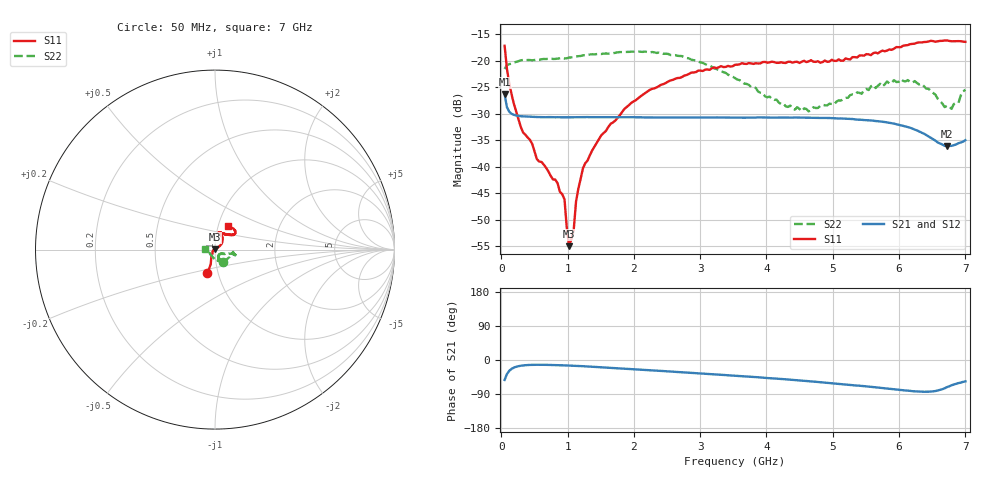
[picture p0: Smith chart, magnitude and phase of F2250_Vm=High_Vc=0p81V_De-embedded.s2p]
! Integrated Device Technology
! Corporate Headquarters
! 6024 Silver Creek Valley Road
! San Jose, CA 95138  USA
! Phone:  1-408-284-8200
! Toll Free:  1-800-223-1366
! Webpage:  http://www.idt.com/
! Timing and RF Division
! 515 Groton Road, Suite 102
! Westford, MA 01886-6024
! Device:  F2250
! Description: Voltage Variable RF Attenuator
! Frequency:  50.0 -  6000.00 MHz
! Package:  3x3 mm Thin QFN Plastic Package: 16 pin
! Ports:  2 RF, 3 DC
!  Pin  1  = GND
!  Pin  2  = NC
!  Pin  3  = RF1  = Port 1
!  Pin  4  = NC
!  Pin  5  = GND
!  Pin  6  = GND
!  Pin  7  = GND
!  Pin  8  = GND
!  Pin  9  = NC
!  Pin 10  = RF2  = Port 2
!  Pin 11  = NC
!  Pin 12  = GND
!  Pin 13  = GND
!  Pin 14  = VCNTRL
!  Pin 15  = VDD
!  Pin 16  = VMODE
! Vcntrl:  0.810 Volts
! Vmode:  +3.300 Volts
! Vdd:  +3.30  Volts
! Current:  1.304 mA
! Data:  The device was measured on a the F2250 evaluation board which has
!  individual transmission lines to the RF pins.  Data was collected
!  using a calibrated network analyzer.  The evaluation board was
!  de-embedded using a TRL calibration technique.
!  The reference plane is the edge of the package pin.
! Misc:  SN 10
!  Action Tracker AT0258
! Date Measured:  2014-11-26
! Date:  2015-10-15  MJV
! Note:
!  Integrated Device Technology supplies this data as a sample of measured
!  data at the package pin for this product.  Your particular data for this
!  product may vary.
!  Data was taken at 25 degrees C.
!  Integrated Device Technology reserves the right to change this data at anytime.
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# GHz S dB R 50
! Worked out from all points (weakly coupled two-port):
!   201 points, 50 MHz to 7 GHz, reference 50 ohm
!   highest |S21| = -26.31 dB at 50 MHz (marker M1); lowest = -36.1 dB at 6.722 GHz (marker M2)
!   lowest |S11| = -55.0 dB at 1.023 GHz (marker M3), VSWR 1.00, Z = 49.9 + j0.141 ohm
!   |S11| at or under -10 dB: start of sweep to end of sweep
!   |S22| runs from -29.5 to -18.2 dB; largest |S21 - S12| = 9.7e-05
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0.05  -17.14 -107.7  -26.31 -52.6  -26.29 -52.5  -21.52 -57.7
0.1195  -24.21 -110.7  -29.59 -28.6  -29.60 -28.6  -20.62 -17.2
0.29325  -32.45 -124.6  -30.45 -15.2  -30.43 -15.2  -19.89 -9.7
0.467  -35.70 -142.9  -30.56 -12.8  -30.56 -12.8  -19.89 -7.8
0.5365  -38.54 -150.8  -30.60 -12.6  -30.58 -12.6  -19.78 -8.6
0.8145  -42.43 171.0  -30.64 -13.4  -30.64 -13.4  -19.62 -11.2
0.9535  -46.15 173.7  -30.66 -14.2  -30.66 -14.2  -19.56 -12.7
0.98825  -51.58 167.9  -30.66 -14.4  -30.66 -14.4  -19.49 -13.0
1.023  -55.00 127.2  -30.66 -14.7  -30.67 -14.7  -19.37 -12.9
1.0925  -51.91 61.6  -30.65 -15.2  -30.65 -15.2  -19.29 -13.3
1.12725  -46.58 46.6  -30.65 -15.4  -30.64 -15.5  -19.16 -13.8
1.2315  -40.30 34.2  -30.63 -16.4  -30.63 -16.4  -18.96 -15.0
1.6485  -31.89 38.6  -30.62 -20.6  -30.63 -20.6  -18.58 -15.7
2.37825  -24.75 45.5  -30.68 -28.5  -30.67 -28.5  -18.42 -15.2
3.525  -20.73 71.1  -30.74 -41.5  -30.72 -41.5  -23.25 -20.4
4.2895  -20.40 75.3  -30.71 -51.0  -30.69 -51.0  -28.57 -38.9
4.7065  -20.15 71.6  -30.74 -56.9  -30.75 -56.9  -28.75 -56.2
5.85325  -17.84 40.2  -31.69 -76.0  -31.71 -76.1  -24.28 -67.2
6.2355  -16.73 38.7  -32.98 -82.6  -32.96 -82.7  -23.81 -76.6
6.722  -16.14 49.0  -36.09 -71.7  -36.12 -71.7  -28.46 -133.5
6.89575  -16.26 56.1  -35.54 -60.9  -35.54 -61.0  -27.93 -170.2
7  -16.40 62.1  -34.97 -56.4  -34.96 -56.5  -25.44 174.6
